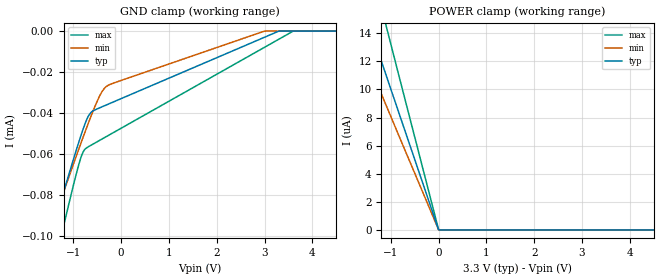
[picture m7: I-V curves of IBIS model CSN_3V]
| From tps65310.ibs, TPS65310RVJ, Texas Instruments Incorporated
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[Model]   CSN_3V
Model_type   Input
Vinl = .8
Vinh = 2.
|   typ   min   max
C_comp   0.01p   0.01p   0.01p
[Voltage Range]   3.3   3   3.6
[Temperature Range]   27   175   -40
[Power Clamp Reference]   3.3   3   3.6
[GND Clamp Reference]   -0   -0   -0
[GND Clamp]
|   Voltage   I(typ)   I(min)   I(max)
-3.3V     -249uA     -222.4uA   -310.6uA
-1.518V   -103.7uA   -99.86uA   -126.9uA
-1.379V   -92.61uA   -90.48uA   -112.9uA
-1.28V    -84.73uA   -83.81uA   -102.9uA
-1.181V   -76.9uA    -77.17uA   -93.07uA
-854.7mV  -52uA      -55.64uA   -62.76uA
-706.2mV  -42.52uA   -46.21uA   -56.85uA
-438.9mV  -37.42uA   -31.2uA    -53.29uA
-240.9mV  -35.44uA   -26.17uA   -50.68uA
2.996V    -3.038uA   -23.42nA   -7.964uA
3.59V     0A         0A         -125.7nA
6.59V     0A         0A         0A
[POWER Clamp]
|   Voltage   I(typ)   I(min)   I(max)
-3.3V     84.74uA    73.95uA    98.41uA
-2.251V   22.56uA    18.19uA    29.82uA
-825mV    8.258uA    6.646uA    10.89uA
-3.3mV    32.39nA    30.52nA    42.87nA
16.5mV    0A         0A         0A
6.59V     0A         0A         0A
